|   stm32f427_437_429_439_lqfp100 IBIS Model
[IBIS ver]   4.2
[File name]  stm32f427_437_429_439_lqfp100.ibs
[File Rev]   1.3
[Date]   05-30-2014
[Source] Data Created at STMicroelectronics
[Notes]   File originated from ELDO simulations.
[Disclaimer]  This information is for modeling purpose only and is
   not guaranted. The information is subject to change without
   notice.
[Copyright] Copyright 2014 STMicroelectronics Inc.
[Component] stm32f427_437_429_439_lqfp100
[Manufacturer] STMicroelectronics
[Package]
| variable   typ   min   max
R_pkg   0.0   NA   NA
L_pkg   0.0H   NA   NA
C_pkg   0.0F   NA   NA
[Pin]   signal_name   model_name   R_pin   L_pin   C_pin
1   PE2   io8p_arsudq_ft   1.324E-01   7.034E-09   1.350E-13
2   PE3   io8p_arsudq_ft   1.333E-01   6.765E-09   1.950E-14
3   PE4   io8p_arsudq_ft   1.290E-01   6.495E-09   1.040E-14
4   PE5   io8p_arsudq_ft   1.253E-01   6.206E-09   5.240E-15
5   PE6   io8p_arsudq_ft   1.205E-01   5.991E-09   7.820E-15
6   VBAT   POWER   1.205E-01   5.950E-09   6.530E-15
7   PC13   io8p_arwsudq_ft_v33   1.179E-01   5.783E-09   6.230E-15
8   PC14   io8p_arwsudq_ft   1.173E-01   5.654E-09   3.110E-15
9   PC15   io8p_arsudq_ft   1.155E-01   5.548E-09   1.390E-15
10   VSS   GND   1.150E-01   5.434E-09   2.920E-15
11   VDD   POWER   1.130E-01   5.296E-09   3.560E-15
12   PH0   io8p_arsudq_ft   1.113E-01   5.231E-09   4.780E-15
13   PH1   io8p_arsudq_ft   1.092E-01   5.142E-09   8.660E-15
14   NRST   ioreset_ft_v33   1.107E-01   5.180E-09   9.030E-15
15   PC0   io8p_ar3wsudq_ft   1.106E-01   5.192E-09   7.980E-15
16   PC1   io8p_ar3wsudq_ft   1.113E-01   5.252E-09   1.030E-14
17   PC2   io8p_ar3wsudq_ft   1.144E-01   5.345E-09   7.000E-15
18   PC3   io8p_ar3wsudq_ft   1.144E-01   5.454E-09   8.650E-15
19   VDD   POWER   1.176E-01   5.621E-09   7.825E-15
20   VREFM   POWER   1.199E-01   5.800E-09   2.290E-16
21   VREFP   POWER   1.223E-01   5.963E-09   1.050E-15
22   VDDA   POWER   1.254E-01   6.187E-09   8.120E-16
23   PA0   io8p_ar3wsudq_ft_v33   1.297E-01   6.485E-09   3.820E-15
24   PA1   io8p_ar3wsudq_ft   1.323E-01   6.715E-09   6.800E-15
25   PA2   io8p_ar3wsudq_ft   1.330E-01   7.014E-09   1.670E-14
26   PA3   io8p_ar3wsudq_ft   1.339E-01   7.050E-09   1.750E-14
27   VSS   GND   1.350E-01   6.804E-09   1.270E-14
28   VDD   POWER   1.305E-01   6.528E-09   9.830E-15
29   PA4   io8p_ar3wsudq_ft   1.254E-01   6.245E-09   6.070E-15
30   PA5   io8p_ar3wsudq_ft   1.250E-01   6.108E-09   5.770E-16
31   PA6   io8p_ar3wsudq_ft   1.218E-01   5.890E-09   1.520E-15
32   PA7   io8p_ar3wsudq_ft   1.191E-01   5.716E-09   5.440E-15
33   PC4   io8p_ar3wsudq_ft   1.164E-01   5.556E-09   4.100E-15
34   PC5   io8p_ar3wsudq_ft   1.133E-01   5.415E-09   3.690E-15
35   PB0   io8p_ar3wsudq_ft   1.127E-01   5.358E-09   3.895E-15
36   PB1   io8p_ar3wsudq_ft   1.123E-01   5.272E-09   1.660E-15
37   PB2   io8p_ar3wsudq_ft   1.118E-01   5.238E-09   7.920E-15
38   PE7   io8p_arsudq_ft   1.110E-01   5.184E-09   9.900E-15
39   PE8   io8p_arsudq_ft   1.146E-01   5.299E-09   7.910E-15
40   PE9   io8p_arsudq_ft   1.145E-01   5.333E-09   7.940E-15
41   PE10   io8p_arsudq_ft   1.154E-01   5.424E-09   4.180E-15
42   PE11   io8p_arsudq_ft   1.170E-01   5.533E-09   6.060E-15
43   PE12   io8p_arsudq_ft   1.202E-01   5.698E-09   5.120E-15
44   PE13   io8p_arsudq_ft   1.226E-01   5.871E-09   4.740E-15
45   PE14   io8p_arsudq_ft   1.263E-01   6.069E-09   1.160E-14
46   PE15   io8p_ar3wsudq_ft   1.297E-01   6.277E-09   9.910E-15
47   PB10   io8p_arsudq_i2cin_ft   1.334E-01   6.508E-09   5.080E-15
48   PB11   io8p_arsudq_i2cin_ft   1.379E-01   6.857E-09   5.470E-15
49   VCAP1   POWER   1.316E-01   6.802E-09   4.180E-15
50   VDD   POWER   1.323E-01   7.042E-09   1.190E-14
51   PB12   io8usb_id_otg_ft   1.318E-01   7.008E-09   1.620E-14
52   PB13   io8usb_vbus_otg_ft   1.318E-01   6.751E-09   2.150E-15
53   PB14   io8usb_lsfs_otg_ft   1.292E-01   6.483E-09   9.175E-15
54   PB15   io8usb_lsfs_otg_ft   1.252E-01   6.202E-09   5.663E-15
55   PD8   io8p_arsudq_ft   1.215E-01   5.986E-09   3.690E-15
56   PD9   io8p_arsudq_ft   1.189E-01   5.807E-09   7.430E-15
57   PD10   io8p_arsudq_ft   1.159E-01   5.635E-09   1.060E-14
58   PD11   io8p_arsudq_ft   1.132E-01   5.471E-09   5.760E-15
59   PD12   io8p_arsudq_ft   1.118E-01   5.354E-09   6.530E-15
60   PD13   io8p_arsudq_ft   1.107E-01   5.276E-09   1.140E-14
61   PD14   io8p_arsudq_ft   1.101E-01   5.204E-09   1.320E-14
62   PD15   io8p_arsudq_ft   1.100E-01   5.180E-09   1.460E-14
63   PC6   io8p_arsudq_ft   1.098E-01   5.154E-09   7.250E-15
64   PC7   io8p_arsudq_ft   1.124E-01   5.258E-09   3.590E-16
65   PC8   io8p_arsudq_ft   1.136E-01   5.332E-09   6.580E-16
66   PC9   io8p_arsudq_i2cin_ft   1.157E-01   5.466E-09   5.085E-16
67   PA8   io8p_arsudq_i2cin_ft   1.170E-01   5.598E-09   5.833E-16
68   PA9   io8usb_vbus_otg_ft   1.190E-01   5.762E-09   5.459E-16
69   PA10   io8usb_id_otg_ft   1.207E-01   5.880E-09   1.390E-14
70   PA11   io8usb_lsfs_otg_ft   1.247E-01   6.108E-09   2.500E-14
71   PA12   io8usb_lsfs_otg_ft   1.244E-01   6.161E-09   3.990E-14
72   PA13   io8p_arsudq_ft   1.302E-01   6.404E-09   3.020E-13
73   VCAP2   POWER   1.351E-01   6.824E-09   1.550E-13
74   VSS   GND   1.394E-01   7.077E-09   1.550E-13
75   VDD   POWER   1.336E-01   7.056E-09   3.900E-14
76   PA14   io8p_arsudq_ft   1.353E-01   7.104E-09   1.630E-14
77   PA15   io8p_arsudq_ft   1.325E-01   6.836E-09   9.760E-15
78   PC10   io8p_arsudq_ft   1.335E-01   6.641E-09   9.300E-15
79   PC11   io8p_arsudq_ft   1.284E-01   6.341E-09   5.420E-15
80   PC12   io8p_arsudq_ft   1.243E-01   6.092E-09   1.180E-15
81   PD0   io8p_arsudq_ft   1.218E-01   5.917E-09   5.460E-15
82   PD1   io8p_arsudq_ft   1.185E-01   5.728E-09   7.000E-15
83   PD2   io8p_arsudq_ft   1.172E-01   5.573E-09   6.060E-15
84   PD3   io8p_arsudq_ft   1.135E-01   5.422E-09   5.450E-15
85   PD4   io8p_arsudq_ft   1.138E-01   5.344E-09   5.290E-16
86   PD5   io8p_arsudq_ft   1.108E-01   5.256E-09   2.990E-15
87   PD6   io8p_arsudq_ft   1.104E-01   5.246E-09   2.060E-15
88   PD7   io8p_arsudq_ft   1.115E-01   5.178E-09   5.680E-15
89   PB3   io8p_arsudq_ft   1.111E-01   5.223E-09   9.910E-15
90   PB4   io8p_arsudq_ft   1.132E-01   5.310E-09   9.050E-15
91   PB5   io8p_ar3wsudq_ft   1.133E-01   5.401E-09   1.290E-14
92   PB6   io8p_arsudq_i2cin_ft   1.158E-01   5.519E-09   1.260E-14
93   PB7   io8p_arsudq_i2cin_ft   1.176E-01   5.673E-09   6.140E-15
94   BOOT0   vpp_test_hv   1.190E-01   5.802E-09   9.370E-15
95   PB8   io8p_arsudq_i2cin_ft   1.219E-01   5.962E-09   7.755E-15
96   PB9   io8p_arsudq_i2cin_ft   1.263E-01   6.158E-09   8.563E-15
97   PE0   io8p_arsudq_ft   1.287E-01   6.367E-09   8.159E-15
98   PE1   io8p_arsudq_ft   1.333E-01   6.700E-09   1.030E-15
99   VSS   GND   1.322E-01   6.844E-09   4.410E-15
100  VDD   POWER   1.323E-01   7.052E-09   1.710E-14
[Diff Pin]   inv_pin   vdiff   tdelay_typ  tdelay_min  tdelay_max
54   53   200mV   NA   NA   NA
71   70   200mV   NA   NA   NA
[Model Selector] io8p_ar3wsudq_ft
io8p00_ar3wsudq_ft_pd_lv  "SPEED00 1P8V, PD=40kOhm"
io8p00_ar3wsudq_ft_pu_lv  "SPEED00 1P8V, PU=40kOhm"
io8p00_ar3wsudq_ft_lv  "SPEED00 1P8V"
io8p01_ar3wsudq_ft_pd_lv  "SPEED01 1P8V, PD=40kOhm"
io8p01_ar3wsudq_ft_pu_lv  "SPEED01 1P8V, PU=40kOhm"
io8p01_ar3wsudq_ft_lv  "SPEED01 1P8V"
io8p10_ar3wsudq_ft_pd_lv  "SPEED10 1P8V, PD=40kOhm"
io8p10_ar3wsudq_ft_pu_lv  "SPEED10 1P8V, PU=40kOhm"
io8p10_ar3wsudq_ft_lv  "SPEED10 1P8V"
io8p11_ar3wsudq_ft_pd_lv  "SPEED11 1P8V, PD=40kOhm"
io8p11_ar3wsudq_ft_pu_lv  "SPEED11 1P8V, PU=40kOhm"
io8p11_ar3wsudq_ft_lv  "SPEED11 1P8V"
io8p00_ar3wsudq_ft_pd  "SPEED00, PD=40kOhm"
io8p00_ar3wsudq_ft_pu  "SPEED00, PU=40kOhm"
io8p00_ar3wsudq_ft  "SPEED00"
io8p01_ar3wsudq_ft_pd  "SPEED01, PD=40kOhm"
io8p01_ar3wsudq_ft_pu  "SPEED01, PU=40kOhm"
io8p01_ar3wsudq_ft  "SPEED01"
io8p10_ar3wsudq_ft_pd  "SPEED10, PD=40kOhm"
io8p10_ar3wsudq_ft_pu  "SPEED10, PU=40kOhm"
io8p10_ar3wsudq_ft  "SPEED10"
io8p11_ar3wsudq_ft_pd  "SPEED11, PD=40kOhm"
io8p11_ar3wsudq_ft_pu  "SPEED11, PU=40kOhm"
io8p11_ar3wsudq_ft  "SPEED11"
[Model Selector] io8p_ar3wsudq_ft_v33
io8p00_ar3wsudq_ft_v33_pd_lv  "SPEED00 1P8V, PD=40kOhm"
io8p00_ar3wsudq_ft_v33_pu_lv  "SPEED00 1P8V, PU=40kOhm"
io8p00_ar3wsudq_ft_v33_lv  "SPEED00 1P8V"
io8p01_ar3wsudq_ft_v33_pd_lv  "SPEED01 1P8V, PD=40kOhm"
io8p01_ar3wsudq_ft_v33_pu_lv  "SPEED01 1P8V, PU=40kOhm"
io8p01_ar3wsudq_ft_v33_lv  "SPEED01 1P8V"
io8p10_ar3wsudq_ft_v33_pd_lv  "SPEED10 1P8V, PD=40kOhm"
io8p10_ar3wsudq_ft_v33_pu_lv  "SPEED10 1P8V, PU=40kOhm"
io8p10_ar3wsudq_ft_v33_lv  "SPEED10 1P8V"
io8p11_ar3wsudq_ft_v33_pd_lv  "SPEED11 1P8V, PD=40kOhm"
io8p11_ar3wsudq_ft_v33_pu_lv  "SPEED11 1P8V, PU=40kOhm"
io8p11_ar3wsudq_ft_v33_lv  "SPEED11 1P8V"
io8p00_ar3wsudq_ft_v33_pd  "SPEED00, PD=40kOhm"
io8p00_ar3wsudq_ft_v33_pu  "SPEED00, PU=40kOhm"
io8p00_ar3wsudq_ft_v33  "SPEED00"
io8p01_ar3wsudq_ft_v33_pd  "SPEED01, PD=40kOhm"
io8p01_ar3wsudq_ft_v33_pu  "SPEED01, PU=40kOhm"
io8p01_ar3wsudq_ft_v33  "SPEED01"
io8p10_ar3wsudq_ft_v33_pd  "SPEED10, PD=40kOhm"
io8p10_ar3wsudq_ft_v33_pu  "SPEED10, PU=40kOhm"
io8p10_ar3wsudq_ft_v33  "SPEED10"
io8p11_ar3wsudq_ft_v33_pd  "SPEED11, PD=40kOhm"
io8p11_ar3wsudq_ft_v33_pu  "SPEED11, PU=40kOhm"
io8p11_ar3wsudq_ft_v33  "SPEED11"
[Model Selector] io8p_arsudq_ft
io8p00_arsudq_ft_pd_lv  "SPEED00 1P8V, PD=40kOhm"
io8p00_arsudq_ft_pu_lv  "SPEED00 1P8V, PU=40kOhm"
io8p00_arsudq_ft_lv  "SPEED00 1P8V"
io8p01_arsudq_ft_pd_lv  "SPEED01 1P8V, PD=40kOhm"
io8p01_arsudq_ft_pu_lv  "SPEED01 1P8V, PU=40kOhm"
io8p01_arsudq_ft_lv  "SPEED01 1P8V"
io8p10_arsudq_ft_pd_lv  "SPEED10 1P8V, PD=40kOhm"
io8p10_arsudq_ft_pu_lv  "SPEED10 1P8V, PU=40kOhm"
io8p10_arsudq_ft_lv  "SPEED10 1P8V"
io8p11_arsudq_ft_pd_lv  "SPEED11 1P8V, PD=40kOhm"
io8p11_arsudq_ft_pu_lv  "SPEED11 1P8V, PU=40kOhm"
io8p11_arsudq_ft_lv  "SPEED11 1P8V"
io8p00_arsudq_ft_pd  "SPEED00, PD=40kOhm"
io8p00_arsudq_ft_pu  "SPEED00, PU=40kOhm"
io8p00_arsudq_ft  "SPEED00"
io8p01_arsudq_ft_pd  "SPEED01, PD=40kOhm"
io8p01_arsudq_ft_pu  "SPEED01, PU=40kOhm"
io8p01_arsudq_ft  "SPEED01"
io8p10_arsudq_ft_pd  "SPEED10, PD=40kOhm"
io8p10_arsudq_ft_pu  "SPEED10, PU=40kOhm"
io8p10_arsudq_ft  "SPEED10"
io8p11_arsudq_ft_pd  "SPEED11, PD=40kOhm"
io8p11_arsudq_ft_pu  "SPEED11, PU=40kOhm"
io8p11_arsudq_ft  "SPEED11"
|[Model Selector] io8p_arsudq_ft_v33
|io8p00_arsudq_ft_v33_pd_lv  "SPEED00 1P8V, PD=40kOhm"
|io8p00_arsudq_ft_v33_pu_lv  "SPEED00 1P8V, PU=40kOhm"
|io8p00_arsudq_ft_v33_lv  "SPEED00 1P8V"
|io8p01_arsudq_ft_v33_pd_lv  "SPEED01 1P8V, PD=40kOhm"
|io8p01_arsudq_ft_v33_pu_lv  "SPEED01 1P8V, PU=40kOhm"
|io8p01_arsudq_ft_v33_lv  "SPEED01 1P8V"
|io8p10_arsudq_ft_v33_pd_lv  "SPEED10 1P8V, PD=40kOhm"
|io8p10_arsudq_ft_v33_pu_lv  "SPEED10 1P8V, PU=40kOhm"
|io8p10_arsudq_ft_v33_lv  "SPEED10 1P8V"
|io8p11_arsudq_ft_v33_pd_lv  "SPEED11 1P8V, PD=40kOhm"
|io8p11_arsudq_ft_v33_pu_lv  "SPEED11 1P8V, PU=40kOhm"
|io8p11_arsudq_ft_v33_lv  "SPEED11 1P8V"
|io8p00_arsudq_ft_v33_pd  "SPEED00, PD=40kOhm"
|io8p00_arsudq_ft_v33_pu  "SPEED00, PU=40kOhm"
|io8p00_arsudq_ft_v33  "SPEED00"
|io8p01_arsudq_ft_v33_pd  "SPEED01, PD=40kOhm"
|io8p01_arsudq_ft_v33_pu  "SPEED01, PU=40kOhm"
|io8p01_arsudq_ft_v33  "SPEED01"
|io8p10_arsudq_ft_v33_pd  "SPEED10, PD=40kOhm"
|io8p10_arsudq_ft_v33_pu  "SPEED10, PU=40kOhm"
|io8p10_arsudq_ft_v33  "SPEED10"
|io8p11_arsudq_ft_v33_pd  "SPEED11, PD=40kOhm"
|io8p11_arsudq_ft_v33_pu  "SPEED11, PU=40kOhm"
|io8p11_arsudq_ft_v33  "SPEED11"
[Model Selector] io8p_arsudq_i2cin_ft
io8p00_arsudq_i2cin_ft_pd_lv  "SPEED00 1P8V, PD=40kOhm"
io8p00_arsudq_i2cin_ft_pu_lv  "SPEED00 1P8V, PU=40kOhm"
io8p00_arsudq_i2cin_ft_lv  "SPEED00 1P8V"
io8p01_arsudq_i2cin_ft_pd_lv  "SPEED01 1P8V, PD=40kOhm"
io8p01_arsudq_i2cin_ft_pu_lv  "SPEED01 1P8V, PU=40kOhm"
io8p01_arsudq_i2cin_ft_lv  "SPEED01 1P8V"
io8p10_arsudq_i2cin_ft_pd_lv  "SPEED10 1P8V, PD=40kOhm"
io8p10_arsudq_i2cin_ft_pu_lv  "SPEED10 1P8V, PU=40kOhm"
io8p10_arsudq_i2cin_ft_lv  "SPEED10 1P8V"
io8p11_arsudq_i2cin_ft_pd_lv  "SPEED11 1P8V, PD=40kOhm"
io8p11_arsudq_i2cin_ft_pu_lv  "SPEED11 1P8V, PU=40kOhm"
io8p11_arsudq_i2cin_ft_lv  "SPEED11 1P8V"
io8p00_arsudq_i2cin_ft_pd  "SPEED00, PD=40kOhm"
io8p00_arsudq_i2cin_ft_pu  "SPEED00, PU=40kOhm"
io8p00_arsudq_i2cin_ft  "SPEED00"
io8p01_arsudq_i2cin_ft_pd  "SPEED01, PD=40kOhm"
io8p01_arsudq_i2cin_ft_pu  "SPEED01, PU=40kOhm"
io8p01_arsudq_i2cin_ft  "SPEED01"
io8p10_arsudq_i2cin_ft_pd  "SPEED10, PD=40kOhm"
io8p10_arsudq_i2cin_ft_pu  "SPEED10, PU=40kOhm"
io8p10_arsudq_i2cin_ft  "SPEED10"
io8p11_arsudq_i2cin_ft_pd  "SPEED11, PD=40kOhm"
io8p11_arsudq_i2cin_ft_pu  "SPEED11, PU=40kOhm"
io8p11_arsudq_i2cin_ft  "SPEED11"
[Model Selector] io8p_arwsudq_ft
io8p00_arwsudq_ft_pd_lv  "SPEED00 1P8V, PD=40kOhm"
io8p00_arwsudq_ft_pu_lv  "SPEED00 1P8V, PU=40kOhm"
io8p00_arwsudq_ft_lv  "SPEED00 1P8V"
io8p01_arwsudq_ft_pd_lv  "SPEED01 1P8V, PD=40kOhm"
io8p01_arwsudq_ft_pu_lv  "SPEED01 1P8V, PU=40kOhm"
io8p01_arwsudq_ft_lv  "SPEED01 1P8V"
io8p10_arwsudq_ft_pd_lv  "SPEED10 1P8V, PD=40kOhm"
io8p10_arwsudq_ft_pu_lv  "SPEED10 1P8V, PU=40kOhm"
io8p10_arwsudq_ft_lv  "SPEED10 1P8V"
io8p11_arwsudq_ft_pd_lv  "SPEED11 1P8V, PD=40kOhm"
io8p11_arwsudq_ft_pu_lv  "SPEED11 1P8V, PU=40kOhm"
io8p11_arwsudq_ft_lv  "SPEED11 1P8V"
io8p00_arwsudq_ft_pd  "SPEED00, PD=40kOhm"
io8p00_arwsudq_ft_pu  "SPEED00, PU=40kOhm"
io8p00_arwsudq_ft  "SPEED00"
io8p01_arwsudq_ft_pd  "SPEED01, PD=40kOhm"
io8p01_arwsudq_ft_pu  "SPEED01, PU=40kOhm"
io8p01_arwsudq_ft  "SPEED01"
io8p10_arwsudq_ft_pd  "SPEED10, PD=40kOhm"
io8p10_arwsudq_ft_pu  "SPEED10, PU=40kOhm"
io8p10_arwsudq_ft  "SPEED10"
io8p11_arwsudq_ft_pd  "SPEED11, PD=40kOhm"
io8p11_arwsudq_ft_pu  "SPEED11, PU=40kOhm"
io8p11_arwsudq_ft  "SPEED11"
[Model Selector] io8p_arwsudq_ft_v33
io8p00_arwsudq_ft_v33_pd_lv  "SPEED00 1P8V, PD=40kOhm"
io8p00_arwsudq_ft_v33_pu_lv  "SPEED00 1P8V, PU=40kOhm"
io8p00_arwsudq_ft_v33_lv  "SPEED00 1P8V"
io8p01_arwsudq_ft_v33_pd_lv  "SPEED01 1P8V, PD=40kOhm"
io8p01_arwsudq_ft_v33_pu_lv  "SPEED01 1P8V, PU=40kOhm"
io8p01_arwsudq_ft_v33_lv  "SPEED01 1P8V"
io8p10_arwsudq_ft_v33_pd_lv  "SPEED10 1P8V, PD=40kOhm"
io8p10_arwsudq_ft_v33_pu_lv  "SPEED10 1P8V, PU=40kOhm"
io8p10_arwsudq_ft_v33_lv  "SPEED10 1P8V"
io8p11_arwsudq_ft_v33_pd_lv  "SPEED11 1P8V, PD=40kOhm"
io8p11_arwsudq_ft_v33_pu_lv  "SPEED11 1P8V, PU=40kOhm"
io8p11_arwsudq_ft_v33_lv  "SPEED11 1P8V"
io8p00_arwsudq_ft_v33_pd  "SPEED00, PD=40kOhm"
io8p00_arwsudq_ft_v33_pu  "SPEED00, PU=40kOhm"
io8p00_arwsudq_ft_v33  "SPEED00"
io8p01_arwsudq_ft_v33_pd  "SPEED01, PD=40kOhm"
io8p01_arwsudq_ft_v33_pu  "SPEED01, PU=40kOhm"
io8p01_arwsudq_ft_v33  "SPEED01"
io8p10_arwsudq_ft_v33_pd  "SPEED10, PD=40kOhm"
io8p10_arwsudq_ft_v33_pu  "SPEED10, PU=40kOhm"
io8p10_arwsudq_ft_v33  "SPEED10"
io8p11_arwsudq_ft_v33_pd  "SPEED11, PD=40kOhm"
io8p11_arwsudq_ft_v33_pu  "SPEED11, PU=40kOhm"
io8p11_arwsudq_ft_v33  "SPEED11"
[Model Selector] io8usb_id_otg_ft
io8p00_id_otg_ft_pd_lv  "SPEED00 1P8V, PD=14kOhm"
io8p00_id_otg_ft_pu_lv  "SPEED00 1P8V, PU=14kOhm"
io8p00_id_otg_ft_lv  "SPEED00 1P8V"
io8p01_id_otg_ft_pd_lv  "SPEED01 1P8V, PD=14kOhm"
io8p01_id_otg_ft_pu_lv  "SPEED01 1P8V, PU=14kOhm"
io8p01_id_otg_ft_lv  "SPEED01 1P8V"
io8p10_id_otg_ft_pd_lv  "SPEED10 1P8V, PD=14kOhm"
io8p10_id_otg_ft_pu_lv  "SPEED10 1P8V, PU=14kOhm"
io8p10_id_otg_ft_lv  "SPEED10 1P8V"
io8p11_id_otg_ft_pd_lv  "SPEED11 1P8V, PD=14kOhm"
io8p11_id_otg_ft_pu_lv  "SPEED11 1P8V, PU=14kOhm"
io8p11_id_otg_ft_lv  "SPEED11 1P8V"
io8p00_id_otg_ft_pd  "SPEED00, PD=14kOhm"
io8p00_id_otg_ft_pu  "SPEED00, PU=14kOhm"
io8p00_id_otg_ft  "SPEED00"
io8p01_id_otg_ft_pd  "SPEED01, PD=14kOhm"
io8p01_id_otg_ft_pu  "SPEED01, PU=14kOhm"
io8p01_id_otg_ft  "SPEED01"
io8p10_id_otg_ft_pd  "SPEED10, PD=14kOhm"
io8p10_id_otg_ft_pu  "SPEED10, PU=14kOhm"
io8p10_id_otg_ft  "SPEED10"
io8p11_id_otg_ft_pd  "SPEED11, PD=14kOhm"
io8p11_id_otg_ft_pu  "SPEED11, PU=14kOhm"
io8p11_id_otg_ft  "SPEED11"
[Model Selector] io8usb_lsfs_otg_ft
io8usb_ls_otg_ft_dpdn_pd  "LS USB DP/DN IO + PD=20kOhm"
io8usb_ls_otg_ft_dpdn_pupu2  "LS USB DP/DN IO + PU/PU2=2.2kOhm"
io8usb_ls_otg_ft_dpdn_pu2  "LS USB DP/DN IO + PU2=1.2kOhm"
io8usb_ls_otg_ft_dpdn_pu  "LS USB DP/DN IO + PU=1.2kOhm"
io8usb_ls_otg_ft_dpdn  "LS USB DP/DN IO"
io8usb_fs_otg_ft_dpdn_pd  "HS USB DP/DN IO + PD=20kOhm"
io8usb_fs_otg_ft_dpdn_pupu2  "HS USB DP/DN IO + PU/PU2=2.2kOhm"
io8usb_fs_otg_ft_dpdn_pu2  "HS USB DP/DN IO + PU2=1.2kOhm"
io8usb_fs_otg_ft_dpdn_pu  "HS USB DP/DN IO + PU=1.2kOhm"
io8usb_fs_otg_ft_dpdn  "HS USB DP/DN IO"
io8p00_lsfs_otg_ft_pd_lv  "SPEED00 1P8V, PD=40kOhm"
io8p00_lsfs_otg_ft_pu_lv  "SPEED00 1P8V, PU=40kOhm"
io8p00_lsfs_otg_ft_lv  "SPEED00 1P8V"
io8p01_lsfs_otg_ft_pd_lv  "SPEED01 1P8V, PD=40kOhm"
io8p01_lsfs_otg_ft_pu_lv  "SPEED01 1P8V, PU=40kOhm"
io8p01_lsfs_otg_ft_lv  "SPEED01 1P8V"
io8p10_lsfs_otg_ft_pd_lv  "SPEED10 1P8V, PD=40kOhm"
io8p10_lsfs_otg_ft_pu_lv  "SPEED10 1P8V, PU=40kOhm"
io8p10_lsfs_otg_ft_lv  "SPEED10 1P8V"
io8p11_lsfs_otg_ft_pd_lv  "SPEED11 1P8V, PD=40kOhm"
io8p11_lsfs_otg_ft_pu_lv  "SPEED11 1P8V, PU=40kOhm"
io8p11_lsfs_otg_ft_lv  "SPEED11 1P8V"
io8p00_lsfs_otg_ft_pd  "SPEED00, PD=40kOhm"
io8p00_lsfs_otg_ft_pu  "SPEED00, PU=40kOhm"
io8p00_lsfs_otg_ft  "SPEED00"
io8p01_lsfs_otg_ft_pd  "SPEED01, PD=40kOhm"
io8p01_lsfs_otg_ft_pu  "SPEED01, PU=40kOhm"
io8p01_lsfs_otg_ft  "SPEED01"
io8p10_lsfs_otg_ft_pd  "SPEED10, PD=40kOhm"
io8p10_lsfs_otg_ft_pu  "SPEED10, PU=40kOhm"
io8p10_lsfs_otg_ft  "SPEED10"
io8p11_lsfs_otg_ft_pd  "SPEED11, PD=40kOhm"
io8p11_lsfs_otg_ft_pu  "SPEED11, PU=40kOhm"
io8p11_lsfs_otg_ft  "SPEED11"
[Model Selector] io8usb_vbus_otg_ft
io8psenb_vbus_otg_ft  "VBUS PULSE, SENSE VB"
io8psenab_vbus_otg_ft  "VBUS PULSE, SENSE VA and VB"
io8psena_vbus_otg_ft  "VBUS PULSE, SENSE VA"
io8psen_vbus_otg_ft  "VBUS PULSE"
io8p00_vbus_otg_ft_pd_lv  "SPEED00 1P8V, PD=40kOhm"
io8p00_vbus_otg_ft_pu_lv  "SPEED00 1P8V, PU=40kOhm"
io8p00_vbus_otg_ft_lv  "SPEED00 1P8V"
io8p01_vbus_otg_ft_pd_lv  "SPEED01 1P8V, PD=40kOhm"
io8p01_vbus_otg_ft_pu_lv  "SPEED01 1P8V, PU=40kOhm"
io8p01_vbus_otg_ft_lv  "SPEED01 1P8V"
io8p10_vbus_otg_ft_pd_lv  "SPEED10 1P8V, PD=40kOhm"
io8p10_vbus_otg_ft_pu_lv  "SPEED10 1P8V, PU=40kOhm"
io8p10_vbus_otg_ft_lv  "SPEED10 1P8V"
io8p11_vbus_otg_ft_pd_lv  "SPEED11 1P8V, PD=40kOhm"
io8p11_vbus_otg_ft_pu_lv  "SPEED11 1P8V, PU=40kOhm"
io8p11_vbus_otg_ft_lv  "SPEED11 1P8V"
io8p00_vbus_otg_ft_pd  "SPEED00, PD=40kOhm"
io8p00_vbus_otg_ft_pu  "SPEED00, PU=40kOhm"
io8p00_vbus_otg_ft  "SPEED00"
io8p01_vbus_otg_ft_pd  "SPEED01, PD=40kOhm"
io8p01_vbus_otg_ft_pu  "SPEED01, PU=40kOhm"
io8p01_vbus_otg_ft  "SPEED01"
io8p10_vbus_otg_ft_pd  "SPEED10, PD=40kOhm"
io8p10_vbus_otg_ft_pu  "SPEED10, PU=40kOhm"
io8p10_vbus_otg_ft  "SPEED10"
io8p11_vbus_otg_ft_pd  "SPEED11, PD=40kOhm"
io8p11_vbus_otg_ft_pu  "SPEED11, PU=40kOhm"
io8p11_vbus_otg_ft  "SPEED11"
[Model Selector] ioreset_ft_v33
ioreset_ft_v33_pu_lv  "ioreset 1P8V + PU=40kOhm"
ioreset_ft_v33_nopu_lv  "ioreset 1P8V"
ioreset_ft_v33_pu  "ioreset + PU=40kOhm"
ioreset_ft_v33_nopu  "ioreset"
[Model Selector] vpp_test_hv
vpp_test_hv_2p4  "Input Buffer 1P8V"
vpp_test_hv_3p3  "Input Buffer"
| Models and submodels in the file (236): io8p00_ar3wsudq_ft_pd_lv (I/O), io8p00_ar3wsudq_ft_pu_lv (I/O), io8p00_ar3wsudq_ft_lv (I/O), io8p01_ar3wsudq_ft_pd_lv (I/O), io8p01_ar3wsudq_ft_pu_lv (I/O), io8p01_ar3wsudq_ft_lv (I/O), io8p10_ar3wsudq_ft_pd_lv (I/O), io8p10_ar3wsudq_ft_pu_lv (I/O), io8p10_ar3wsudq_ft_lv (I/O), io8p11_ar3wsudq_ft_pd_lv (I/O), io8p11_ar3wsudq_ft_pu_lv (I/O), io8p11_ar3wsudq_ft_lv (I/O), io8p00_ar3wsudq_ft_pd (I/O), io8p00_ar3wsudq_ft_pu (I/O), io8p00_ar3wsudq_ft (I/O), io8p01_ar3wsudq_ft_pd (I/O), io8p01_ar3wsudq_ft_pu (I/O), io8p01_ar3wsudq_ft (I/O), io8p10_ar3wsudq_ft_pd (I/O), io8p10_ar3wsudq_ft_pu (I/O), io8p10_ar3wsudq_ft (I/O), io8p11_ar3wsudq_ft_pd (I/O), io8p11_ar3wsudq_ft_pu (I/O), io8p11_ar3wsudq_ft (I/O), io8p00_ar3wsudq_ft_v33_pd_lv (I/O), io8p00_ar3wsudq_ft_v33_pu_lv (I/O), io8p00_ar3wsudq_ft_v33_lv (I/O), io8p01_ar3wsudq_ft_v33_pd_lv (I/O), io8p01_ar3wsudq_ft_v33_pu_lv (I/O), io8p01_ar3wsudq_ft_v33_lv (I/O), io8p10_ar3wsudq_ft_v33_pd_lv (I/O), io8p10_ar3wsudq_ft_v33_pu_lv (I/O), io8p10_ar3wsudq_ft_v33_lv (I/O), io8p11_ar3wsudq_ft_v33_pd_lv (I/O), io8p11_ar3wsudq_ft_v33_pu_lv (I/O), io8p11_ar3wsudq_ft_v33_lv (I/O), io8p00_ar3wsudq_ft_v33_pd (I/O), io8p00_ar3wsudq_ft_v33_pu (I/O), io8p00_ar3wsudq_ft_v33 (I/O), io8p01_ar3wsudq_ft_v33_pd (I/O), io8p01_ar3wsudq_ft_v33_pu (I/O), io8p01_ar3wsudq_ft_v33 (I/O), io8p10_ar3wsudq_ft_v33_pd (I/O), io8p10_ar3wsudq_ft_v33_pu (I/O), io8p10_ar3wsudq_ft_v33 (I/O), io8p11_ar3wsudq_ft_v33_pd (I/O), io8p11_ar3wsudq_ft_v33_pu (I/O), io8p11_ar3wsudq_ft_v33 (I/O), io8p00_arsudq_ft_pd_lv (I/O), io8p00_arsudq_ft_pu_lv (I/O), io8p00_arsudq_ft_lv (I/O), io8p01_arsudq_ft_pd_lv (I/O), io8p01_arsudq_ft_pu_lv (I/O), io8p01_arsudq_ft_lv (I/O), io8p10_arsudq_ft_pd_lv (I/O), io8p10_arsudq_ft_pu_lv (I/O), io8p10_arsudq_ft_lv (I/O), io8p11_arsudq_ft_pd_lv (I/O), io8p11_arsudq_ft_pu_lv (I/O), io8p11_arsudq_ft_lv (I/O), io8p00_arsudq_ft_pd (I/O), io8p00_arsudq_ft_pu (I/O), io8p00_arsudq_ft (I/O), io8p01_arsudq_ft_pd (I/O), io8p01_arsudq_ft_pu (I/O), io8p01_arsudq_ft (I/O), io8p10_arsudq_ft_pd (I/O), io8p10_arsudq_ft_pu (I/O), io8p10_arsudq_ft (I/O), io8p11_arsudq_ft_pd (I/O), io8p11_arsudq_ft_pu (I/O), io8p11_arsudq_ft (I/O), io8p00_arsudq_i2cin_ft_pd_lv (I/O), io8p00_arsudq_i2cin_ft_pu_lv (I/O), io8p00_arsudq_i2cin_ft_lv (I/O), io8p01_arsudq_i2cin_ft_pd_lv (I/O), io8p01_arsudq_i2cin_ft_pu_lv (I/O), io8p01_arsudq_i2cin_ft_lv (I/O), io8p10_arsudq_i2cin_ft_pd_lv (I/O), io8p10_arsudq_i2cin_ft_pu_lv (I/O)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
